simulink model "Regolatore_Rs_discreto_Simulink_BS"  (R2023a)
settings: Solver=VariableStepAuto  StartTime=0.0  StopTime=10.0  RelTol=1e-3
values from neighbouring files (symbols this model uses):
  grs = (1+tau1*s)/(1+tau2*s)    [Regolatore_Rs_discreto_Simulink.m]
  grz = (a*z+b)/(c*z+d)    [Regolatore_Rs_discreto_Simulink.m]
  gs = 25/((s+1)^2+4)    [Campionamento_ideale.m]    (also in Regolatore_K_discreto.m = 25/(s*(s+1)*(s+10)); Regolatore_Rs_discreto_Simulink.m = 25/(s*(s+1)*(s+10)))
  Par = [a b c d]    [Regolatore_Rs_discreto_Simulink.m]
  Port = 1    [Regolatore_Rs_discreto_Simulink.m]
  T = 0.4    [Campionamento_ideale.m]    (also in Regolatore_Rs_discreto_Simulink.m = T_Range(ii))
  Ts = T    [Regolatore_Rs_discreto_Simulink.m]

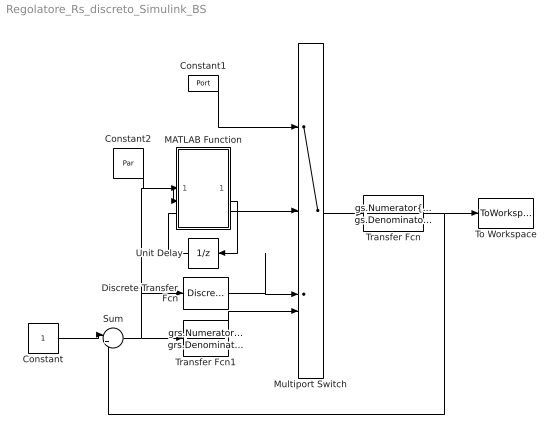
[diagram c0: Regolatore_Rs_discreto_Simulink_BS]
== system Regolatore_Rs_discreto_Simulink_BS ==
  Constant : Constant
  Constant1 : Constant  Value=Port
  Constant2 : Constant  Value=Par
  Discrete Transfer Fcn : DiscreteTransferFcn  Numerator=grz.Numerator{1}  Denominator=grz.Denominator{1}  SampleTime=T
  MATLAB Function : MATLAB Function  TreatAsAtomicUnit=on  SystemSampleTime=T
  Multiport Switch : MultiPortSwitch
  Sum : Sum  Inputs=|+-
  To Workspace : ToWorkspace  VariableName=y  SaveFormat=Timeseries  SampleTime=Ts
  Transfer Fcn : TransferFcn  Numerator=gs.Numerator{1}  Denominator=gs.Denominator{1}
  Transfer Fcn1 : TransferFcn  Numerator=grs.Numerator{1}  Denominator=grs.Denominator{1}
  Unit Delay : UnitDelay  InitialCondition=[0 0]  SampleTime=T  HasFrameUpgradeWarning=on
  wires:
  Constant/1 -> Sum/1
  Transfer Fcn/1 -> To Workspace/1, Sum/2
  Sum/1 -> Transfer Fcn1/1, Discrete Transfer Fcn/1, MATLAB Function/2(e_k)
  Multiport Switch/1 -> Transfer Fcn/1
  Transfer Fcn1/1 -> Multiport Switch/4
  Constant1/1 -> Multiport Switch/1
  Discrete Transfer Fcn/1 -> Multiport Switch/3
  MATLAB Function/1(m_k) -> Multiport Switch/2
  MATLAB Function/2(x_k) -> Unit Delay/1
  Unit Delay/1 -> MATLAB Function/3(x_km1)
  Constant2/1 -> MATLAB Function/1(Par)

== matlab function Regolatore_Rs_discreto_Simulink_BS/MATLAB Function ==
function [m_k, x_k] = fcn(Par,e_k,x_km1)
%%% Equazione alle differenze:
%%%         m_k=(-d*m_km1+a*e_k+b*e_km1)/c
%%% Parametri dell'equazione alle differenze
a=Par(1);
b=Par(2);
c=Par(3);
d=Par(4);
%%%  Vettore di stato del sistema all'istante k-1
e_km1=x_km1(1);
m_km1=x_km1(2);
%%%  Equazione alle differenze
m_k=(-d*m_km1+a*e_k+b*e_km1)/c;
%%%  Vettore di stato del sistema all'istante k
x_k=[e_k; m_k];
